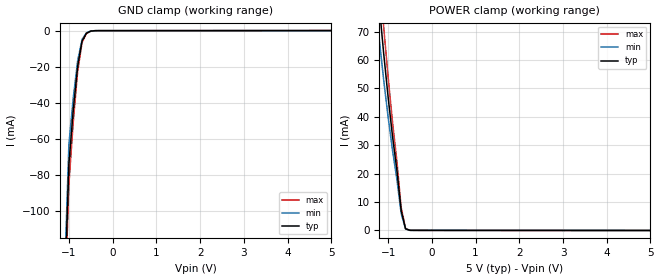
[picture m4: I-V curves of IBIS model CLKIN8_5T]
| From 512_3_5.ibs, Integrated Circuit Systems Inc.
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|   0.8 um mask 5.0V  INPUT  Model
| This model is suitable for CLK INPUT Pin (TTL level) on the
|0.8 um mask
[Model]   CLKIN8_5T
Model_type   Input
Vinl=0.8V   |  Input logic "low" DC voltage
Vinh=2.0V   |  Input logic "high" DC voltage
|   typ   min   max
C_comp   5pF   4pF   6pF
|   typ   min   max
[Voltage range]  5.0V   4.5V   5.5V
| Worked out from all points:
|   GND clamp passes 1 mA (typ) near -0.56 V on its own axis
|   POWER clamp passes 1 mA (typ) near -0.61 V on its own axis
[GND_clamp]
|Voltage I (typ)   I (min)   I (max)
-5V       -3A        -3A        -3A
-1V       -74.28mA   -63.14mA   -85.43mA
-900mV    -43.97mA   -37.37mA   -50.56mA
-800mV    -19.88mA   -16.9mA    -22.86mA
-700mV    -5.86mA    -4.98mA    -6.74mA
-600mV    -1.45mA    -1.23mA    -1.67mA
-500mV    -270uA     -230uA     -310uA
-400mV    -35.1uA    -30uA      -40uA
5V        18.1uA     15.4uA     20.8uA
[POWER_clamp]
|Voltage I (typ)   I (min)   I (max)
-5V       3A         3A         3A
-1.3V     98.74mA    83.93mA    113.6mA
-1.2V     78.97mA    67.13mA    90.82mA
-1.1V     62.22mA    52.89mA    71.56mA
-1V       47.09mA    40.03mA    54.16mA
-900mV    33.36mA    28.35mA    38.36mA
-800mV    21.36mA    18.16mA    24.57mA
-700mV    6.943mA    5.902mA    7.984mA
-600mV    566uA      481uA      651uA
-500mV    41uA       34.9uA     47.2uA
-400mV    23.2uA     19.7uA     26.6uA
5V        -17.4uA    -15uA      -20uA
